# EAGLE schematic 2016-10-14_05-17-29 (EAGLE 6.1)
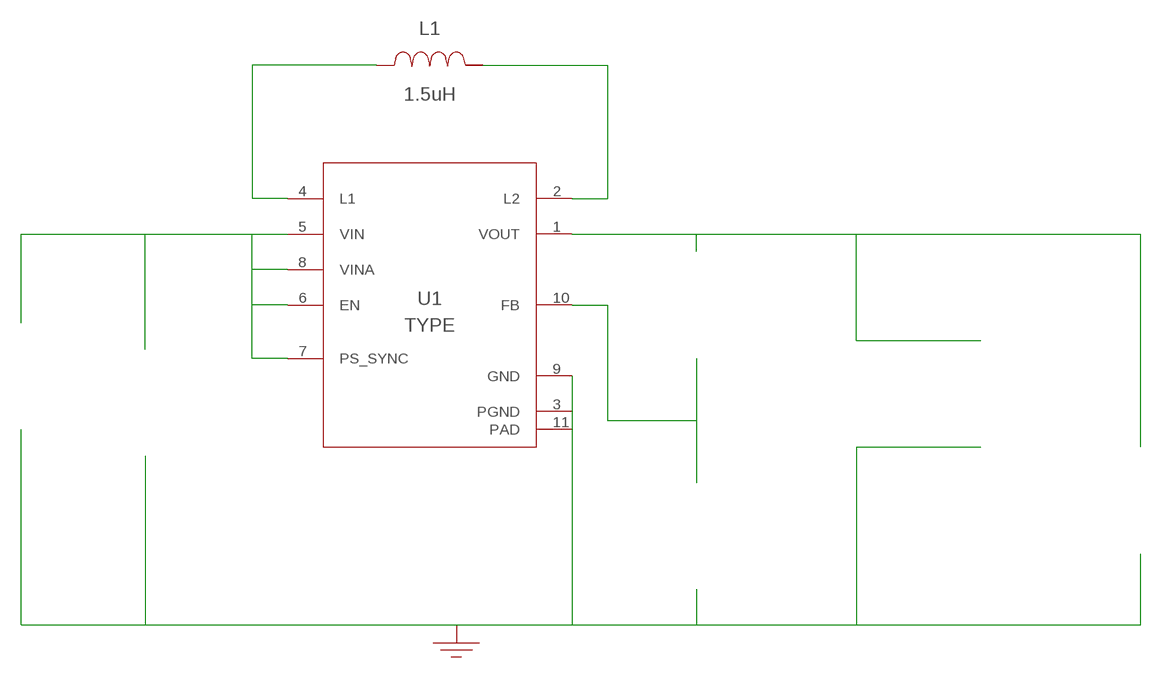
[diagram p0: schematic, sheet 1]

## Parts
CIN  10uF  LMK212BJ106KG-TLMK212BJ106KG-T  [0805]  (not placed on a sheet)
COUT  22uF  LMK212BJ226MG-TLMK212BJ226MG-T  [0805]  (not placed on a sheet)
COUT_2  22uF  LMK212BJ226MG-TLMK212BJ226MG-T  [0805]  (not placed on a sheet)
GND  WB_GND  WB_GNDWB_GND  [WB_GND]
L1  1.5uH  LQM21PN1R5MC0DLQM21PN1R5MC0D  [0805]
RFBB  178k  CRCW0402178KFKEDCRCW0402178KFKED  [0402]  (not placed on a sheet)
RFBT  1M  CRCW04021M00FKEDCRCW04021M00FKED  [0402]  (not placed on a sheet)
RLOAD  WB_LOAD_RESISTOR  WB_LOAD_RESISTORWB_LOAD_RESISTOR  [WB_LOAD_RESISTOR]  (not placed on a sheet)
U1  TPS63000DRCR  TPS63000DRCRTPS63000DRCR  [DRC0010J]
VIN  WB_STARTUP_VOLTAGE_SOURCE  WB_STARTUP_VOLTAGE_SOURCEWB_STARTUP_VOLTAGE_SOURCE  [WB_STARTUP_VOLTAGE_SOURCE]  (not placed on a sheet)

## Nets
0: Cin.2@2 Cout.2@2 Cout_2.2@2 GND.1 Rfbb.2@2 Rload.2@2 U1.3(PGND) U1.9(GND) U1.11(PAD) Vin.-@2
1: Cin.1@1 U1.5(VIN) U1.6(EN) U1.7(PS_SYNC) U1.8(VINA) Vin.+@1
2: L1.1 U1.4(L1)
3: Rfbb.1@1 Rfbt.2@2 U1.10(FB)
4: L1.2 U1.2(L2)
6: Cout.1@1 Cout_2.1@1 Rfbt.1@1 Rload.1@1 U1.1(VOUT)
Unconnected: CIN.1 CIN.2 COUT.1 COUT.2 COUT_2.1 COUT_2.2 RFBB.1 RFBB.2 RFBT.1 RFBT.2 RLOAD.1 RLOAD.2 VIN.1(+) VIN.2(-)

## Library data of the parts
CIN = AcceleratedDesigns_Lib:LMK212BJ106KG-T; Cap: 1.0E-5; ESR: 0.0; IRMS: 0.0; Manufacturer_Name: Taiyo Yuden; Manufacturer_Part_Number: LMK212BJ106KG-T; VDC: 10.0; Vendor: Taiyo Yuden
COUT COUT_2 = AcceleratedDesigns_Lib:LMK212BJ226MG-T; Cap: 2.2E-5; ESR: 0.0; IRMS: 0.0; Manufacturer_Name: Taiyo Yuden; Manufacturer_Part_Number: LMK212BJ226MG-T; VDC: 10.0; Vendor: Taiyo Yuden
GND = AcceleratedDesigns_Lib:WB_GND; Manufacturer_Name: WB_GND; Manufacturer_Part_Number: WB_GND; PowerPortType: POWER_GROUND; Value: Value
L1 = AcceleratedDesigns_Lib:LQM21PN1R5MC0D; DCR: 0.26; IDC: 0.7; L: 1.5E-6; Manufacturer_Name: MuRata; Manufacturer_Part_Number: LQM21PN1R5MC0D; Vendor: MuRata
RFBB = AcceleratedDesigns_Lib:CRCW0402178KFKED; Manufacturer_Name: Vishay-Dale; Manufacturer_Part_Number: CRCW0402178KFKED; Power: 0.063; Resistance: 178000.0; Tolerance: 1.0; Vendor: Vishay-Dale
RFBT = AcceleratedDesigns_Lib:CRCW04021M00FKED; Manufacturer_Name: Vishay-Dale; Manufacturer_Part_Number: CRCW04021M00FKED; Power: 0.063; Resistance: 1000000.0; Tolerance: 1.0; Vendor: Vishay-Dale
RLOAD = AcceleratedDesigns_Lib:WB_LOAD_RESISTOR; Manufacturer_Name: WB_LOAD_RESISTOR; Manufacturer_Part_Number: WB_LOAD_RESISTOR; PowerPortType: POWER_GROUND; Value: Value
U1 = AcceleratedDesigns_Lib:TPS63000DRCR; CompType: IC; Manufacturer: Texas Instruments; Manufacturer_Name: Texas Instruments; Manufacturer_Part_Number: TPS63000DRCR; MountType: SMT; PIN_COUNT: 11; PackageReference: DRC0010A; PartNumber: TPS63000DRC; RefDes: RefDes; RoHS: Y; TYPE: TYPE; Value: Value
VIN = AcceleratedDesigns_Lib:WB_STARTUP_VOLTAGE_SOURCE; Manufacturer_Name: WB_STARTUP_VOLTAGE_SOURCE; Manufacturer_Part_Number: WB_STARTUP_VOLTAGE_SOURCE; PowerPortType: POWER_GROUND; Value: Value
